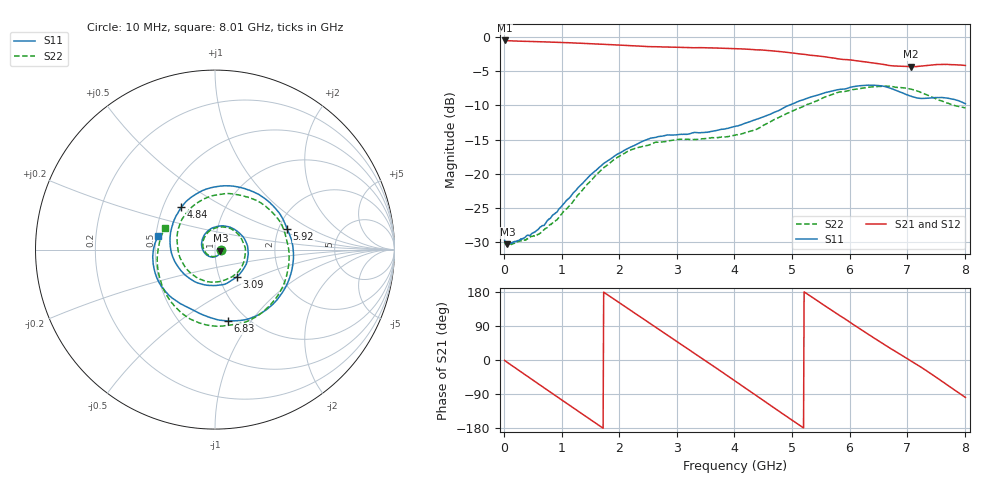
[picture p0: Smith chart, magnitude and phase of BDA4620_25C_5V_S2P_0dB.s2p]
!Agilent Technologies,E5071B,MY42404982,A.09.10
!Date: Wed May 06 08:58:03 2026
!Data & Calibration Information:
!Freq	S11:SOLT2(ON)	S21:SOLT2(ON)	S12:SOLT2(ON)	S22:SOLT2(ON)
# Hz S RI R 50
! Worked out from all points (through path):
!   801 points, 10 MHz to 8.01 GHz, reference 50 ohm
!   highest |S21| = -0.45 dB at 10 MHz (marker M1); lowest = -4.3 dB at 7.06 GHz (marker M2)
!   group delay of S21, straight-line fit = 284 ps
!   lowest |S11| = -30.4 dB at 60 MHz (marker M3), VSWR 1.06, Z = 53.1 - j0.534 ohm
!   |S11| at or under -10 dB: start of sweep to 4.938 GHz
!   |S22| runs from -30.7 to -7.2 dB; largest |S21 - S12| = 0.004
!   S11 on the Smith chart (normalised r, x): 10 MHz: 1.07, -0.01; 3.09 GHz: 1.21, -0.38; 4.84 GHz: 0.62, +0.32; 5.92 GHz: 2.23, +0.62; 6.83 GHz: 0.82, -0.78; 8.01 GHz: 0.51, +0.09
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1e7  0.0322 -0.00239  0.9488 -0.0203  0.9501 -0.0204  0.031 -0.0019
6e7  0.0299 -0.00502  0.9387 -0.1084  0.9406 -0.1098  0.0293 -0.00322
3.7e8  0.0223 -0.0259  0.7246 -0.5916  0.7249 -0.593  0.0241 -0.0222
7.3e8  -0.0133 -0.0416  0.2083 -0.9016  0.2081 -0.9033  -0.00645 -0.0392
1.03e9  -0.0559 -0.0213  -0.2877 -0.8696  -0.2886 -0.8703  -0.047 -0.0231
1.35e9  -0.0743 0.039  -0.7099 -0.5612  -0.7101 -0.5618  -0.0679 0.0315
1.93e9  0.0308 0.1321  -0.8188 0.3238  -0.8197 0.3247  0.0248 0.1258
2.32e9  0.1394 0.0893  -0.4093 0.7619  -0.411 0.7627  0.129 0.0865
2.68e9  0.1854 -0.0245  0.1217 0.8435  0.1231 0.8446  0.1695 -0.0121
3.09e9  0.1199 -0.1527  0.6481 0.543  0.6504 0.5425  0.1228 -0.1296
3.54e9  -0.0286 -0.1999  0.8319 -0.0929  0.8332 -0.094  -0.0132 -0.1812
4.01e9  -0.184 -0.1237  0.4711 -0.6795  0.4705 -0.6812  -0.1598 -0.1058
4.42e9  -0.25 0.0387  -0.1127 -0.8014  -0.1144 -0.8014  -0.2114 0.0432
4.84e9  -0.187 0.2364  -0.6168 -0.4809  -0.6177 -0.4812  -0.1379 0.2284
5.35e9  0.0996 0.3538  -0.7138 0.1836  -0.7149 0.1844  0.1279 0.3053
5.92e9  0.4024 0.1146  -0.2163 0.6518  -0.2174 0.6527  0.395 0.0694
6.27e9  0.4166 -0.1554  0.1907 0.6328  0.1914 0.633  0.3921 -0.1693
6.68e9  0.1827 -0.3871  0.5211 0.341  0.5225 0.3417  0.1934 -0.3933
6.83e9  0.0728 -0.3973  0.5803 0.2047  0.5819 0.2045  0.084 -0.4206
7.06e9  -0.0645 -0.3653  0.6093 -0.0233  0.611 -0.024  -0.0882 -0.4082
7.61e9  -0.3102 -0.186  0.3452 -0.5307  0.346 -0.5318  -0.3157 -0.1256
8.01e9  -0.3164 0.0772  -0.0948 -0.6147  -0.0952 -0.6159  -0.2776 0.1214
